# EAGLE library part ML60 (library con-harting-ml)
3M
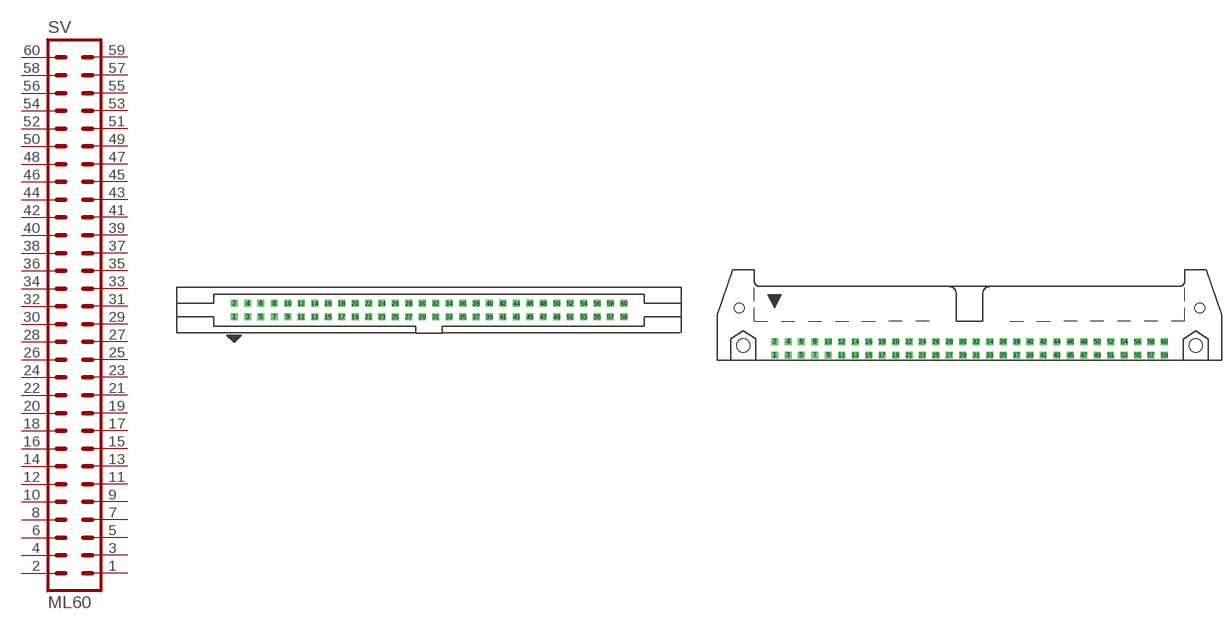
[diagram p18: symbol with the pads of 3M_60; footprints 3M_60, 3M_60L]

Designator prefix SV

## ML603M (OC_FARNELL: unknown; OC_NEWARK: unknown)  [3M_60]
1  1  pas
2  2  pas
3  3  pas
4  4  pas
5  5  pas
6  6  pas
7  7  pas
8  8  pas
9  9  pas
10  10  pas
11  11  pas
12  12  pas
13  13  pas
14  14  pas
15  15  pas
16  16  pas
17  17  pas
18  18  pas
19  19  pas
20  20  pas
21  21  pas
22  22  pas
23  23  pas
24  24  pas
25  25  pas
26  26  pas
27  27  pas
28  28  pas
29  29  pas
30  30  pas
31  31  pas
32  32  pas
33  33  pas
34  34  pas
35  35  pas
36  36  pas
37  37  pas
38  38  pas
39  39  pas
40  40  pas
41  41  pas
42  42  pas
43  43  pas
44  44  pas
45  45  pas
46  46  pas
47  47  pas
48  48  pas
49  49  pas
50  50  pas
51  51  pas
52  52  pas
53  53  pas
54  54  pas
55  55  pas
56  56  pas
57  57  pas
58  58  pas
59  59  pas
60  60  pas

## ML603ML (OC_FARNELL: unknown; OC_NEWARK: unknown)  [3M_60L]
Pads as for 3M_60

## Footprint 3M_60 (pad centres in mm)
3M
drill 0.813 square: 1 -36.83,-1.27; 2 -36.83,1.27; 3 -34.29,-1.27; 4 -34.29,1.27; 5 -31.75,-1.27; 6 -31.75,1.27; 7 -29.21,-1.27; 8 -29.21,1.27; 9 -26.67,-1.27; 10 -26.67,1.27; 11 -24.13,-1.27; 12 -24.13,1.27; 13 -21.59,-1.27; 14 -21.59,1.27; 15 -19.05,-1.27; 16 -19.05,1.27; 17 -16.51,-1.27; 18 -16.51,1.27; 19 -13.97,-1.27; 20 -13.97,1.27; 21 -11.43,-1.27; 22 -11.43,1.27; 23 -8.89,-1.27; 24 -8.89,1.27; 25 -6.35,-1.27; 26 -6.35,1.27; 27 -3.81,-1.27; 28 -3.81,1.27; 29 -1.27,-1.27; 30 -1.27,1.27; 31 1.27,-1.27; 32 1.27,1.27; 33 3.81,-1.27; 34 3.81,1.27; 35 6.35,-1.27; 36 6.35,1.27; 37 8.89,-1.27; 38 8.89,1.27; 39 11.43,-1.27; 40 11.43,1.27; 41 13.97,-1.27; 42 13.97,1.27; 43 16.51,-1.27; 44 16.51,1.27; 45 19.05,-1.27; 46 19.05,1.27; 47 21.59,-1.27; 48 21.59,1.27; 49 24.13,-1.27; 50 24.13,1.27; 51 26.67,-1.27; 52 26.67,1.27; 53 29.21,-1.27; 54 29.21,1.27; 55 31.75,-1.27; 56 31.75,1.27; 57 34.29,-1.27; 58 34.29,1.27; 59 36.83,-1.27; 60 36.83,1.27

## Footprint 3M_60L (pad centres in mm)
3M
drill 0.813 square: 1 -36.83,-5.08; 2 -36.83,-2.54; 3 -34.29,-5.08; 4 -34.29,-2.54; 5 -31.75,-5.08; 6 -31.75,-2.54; 7 -29.21,-5.08; 8 -29.21,-2.54; 9 -26.67,-5.08; 10 -26.67,-2.54; 11 -24.13,-5.08; 12 -24.13,-2.54; 13 -21.59,-5.08; 14 -21.59,-2.54; 15 -19.05,-5.08; 16 -19.05,-2.54; 17 -16.51,-5.08; 18 -16.51,-2.54; 19 -13.97,-5.08; 20 -13.97,-2.54; 21 -11.43,-5.08; 22 -11.43,-2.54; 23 -8.89,-5.08; 24 -8.89,-2.54; 25 -6.35,-5.08; 26 -6.35,-2.54; 27 -3.81,-5.08; 28 -3.81,-2.54; 29 -1.27,-5.08; 30 -1.27,-2.54; 31 1.27,-5.08; 32 1.27,-2.54; 33 3.81,-5.08; 34 3.81,-2.54; 35 6.35,-5.08; 36 6.35,-2.54; 37 8.89,-5.08; 38 8.89,-2.54; 39 11.43,-5.08; 40 11.43,-2.54; 41 13.97,-5.08; 42 13.97,-2.54; 43 16.51,-5.08; 44 16.51,-2.54; 45 19.05,-5.08; 46 19.05,-2.54; 47 21.59,-5.08; 48 21.59,-2.54; 49 24.13,-5.08; 50 24.13,-2.54; 51 26.67,-5.08; 52 26.67,-2.54; 53 29.21,-5.08; 54 29.21,-2.54; 55 31.75,-5.08; 56 31.75,-2.54; 57 34.29,-5.08; 58 34.29,-2.54; 59 36.83,-5.08; 60 36.83,-2.54
hole 2.54 at -42.748,-3.277
hole 2.54 at 42.748,-3.277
